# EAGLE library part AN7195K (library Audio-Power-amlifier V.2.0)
The AN7195K is an audio power IC developed for the sound output of car audio (dual 15 W). It is incorporating various protection circuits to protect the IC from destruction by GND-open short-circuit to GND and power supply surge which are the most important subjects of power IC protection, and the IC will largely
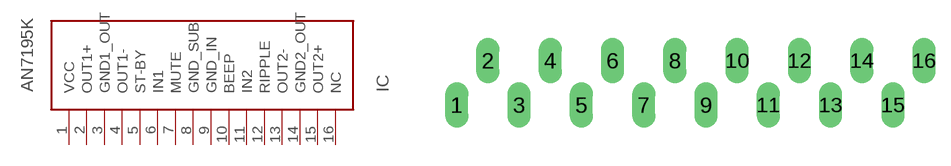
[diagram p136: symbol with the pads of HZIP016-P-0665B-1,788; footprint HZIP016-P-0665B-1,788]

Designator prefix IC

## AN7195K  [HZIP016-P-0665B-1,788]
1  VCC  pwr
2  OUT1+  out
3  GND1_OUT  pwr
4  OUT1-  out
5  ST-BY  in
6  IN1  in
7  MUTE  in
8  GND_SUB  pwr
9  GND_IN  pwr
10  BEEP  in
11  IN2  in
12  RIPPLE
13  OUT2-  out
14  GND2_OUT  pwr
15  OUT2+  out
16  NC  nc

## Footprint HZIP016-P-0665B-1,788 (pad centres in mm)
drill 0.8 long: 1 -13.334,0; 2 -11.556,2.539; 3 -9.778,-0.001; 4 -8,2.539; 5 -6.222,-0.001; 6 -4.444,2.539; 7 -2.666,0; 8 -0.888,2.539; 9 0.889,-0.001; 10 2.668,2.538; 11 4.446,0; 12 6.224,2.539; 13 8,-0.001; 14 9.78,2.539; 15 11.557,-0.001; 16 13.337,2.539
